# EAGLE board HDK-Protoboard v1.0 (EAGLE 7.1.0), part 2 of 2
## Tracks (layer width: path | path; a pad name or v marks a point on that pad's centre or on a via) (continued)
N$793  (via drill 0.89 pad 1.65)
  other vias: 63.88,62.87
N$794  (via drill 0.89 pad 1.65)
  other vias: 61.34,62.87
N$795  (via drill 0.89 pad 1.65)
  other vias: 63.88,60.33
N$796  (via drill 0.89 pad 1.65)
  other vias: 66.42,60.33
N$797  (via drill 0.89 pad 1.65)
  other vias: 63.88,57.79
N$798  (via drill 0.89 pad 1.65)
  other vias: 64.01,55.25
N$799  (via drill 0.89 pad 1.65)
  other vias: 66.42,55.25
N$800  (via drill 0.89 pad 1.65)
  other vias: 63.88,52.71
N$801  (via drill 0.89 pad 1.65)
  other vias: 61.34,52.71
N$802  (via drill 0.89 pad 1.65)
  other vias: 63.88,50.17
N$803  (via drill 0.89 pad 1.65)
  other vias: 66.42,50.17
N$804  (via drill 0.89 pad 1.65)
  other vias: 63.88,47.63
N$805  (via drill 0.89 pad 1.65)
  other vias: 61.34,47.63
N$806  (via drill 0.89 pad 1.65)
  other vias: 63.88,45.09
N$807  (via drill 0.89 pad 1.65)
  other vias: 66.42,45.09
N$808  (via drill 0.89 pad 1.65)
  other vias: 61.34,42.55
N$809  (via drill 0.89 pad 1.65)
  other vias: 63.88,42.55
N$810  (via drill 0.89 pad 1.65)
  other vias: 63.88,40.01
N$811  (via drill 0.89 pad 1.65)
  other vias: 66.42,40.01
N$812  (via drill 0.89 pad 1.65)
  other vias: 63.88,37.47
N$813  (via drill 0.89 pad 1.65)
  other vias: 63.88,34.93
N$814  (via drill 0.89 pad 1.65)
  other vias: 66.42,34.93
N$815  (via drill 0.89 pad 1.65)
  other vias: 61.34,32.39
N$816  (via drill 0.89 pad 1.65)
  other vias: 63.88,32.39
N$817  (via drill 0.89 pad 1.65)
  other vias: 63.88,29.85
N$818  (via drill 0.89 pad 1.65)
  other vias: 66.42,29.85
N$819  (via drill 0.89 pad 1.65)
  other vias: 61.34,27.31
N$820  (via drill 0.89 pad 1.65)
  other vias: 63.88,27.31
N$821  (via drill 0.89 pad 1.65)
  other vias: 63.88,24.77
N$822  (via drill 0.89 pad 1.65)
  other vias: 66.42,24.77
N$823  (via drill 0.89 pad 1.65)
  other vias: 61.34,22.23
N$824  (via drill 0.89 pad 1.65)
  other vias: 63.88,22.23
N$825  (via drill 0.89 pad 1.65)
  other vias: 63.88,19.69
N$826  (via drill 0.89 pad 1.65)
  other vias: 66.42,19.69
N$827  (via drill 0.89 pad 1.65)
  other vias: 61.34,17.15
N$828  (via drill 0.89 pad 1.65)
  other vias: 63.88,17.15
N$829  (via drill 0.89 pad 1.65)
  other vias: 61.34,12.07
N$830  (via drill 0.89 pad 1.65)
  other vias: 63.88,12.07
N$831  (via drill 0.89 pad 1.65)
  other vias: 63.88,14.61
N$832  (via drill 0.89 pad 1.65)
  other vias: 66.42,14.61
N$833  (via drill 0.89 pad 1.65)
  other vias: 63.88,9.53
N$834  (via drill 0.89 pad 1.65)
  other vias: 66.42,9.53
N$835  (via drill 0.89 pad 1.65)
  other vias: 61.34,6.99
N$836  (via drill 0.89 pad 1.65)
  other vias: 63.88,6.99
N$837  (via drill 0.89 pad 1.65)
  other vias: 63.88,4.45
N$838  (via drill 0.89 pad 1.65)
  other vias: 66.42,4.45
N$839  (via drill 0.89 pad 1.65)
  other vias: 61.34,1.91
N$840  (via drill 0.89 pad 1.65)
  other vias: 63.88,1.91
N$841
  Top 0.406: 43.56,9.53 43.56,1.91
N$842  (via drill 0.89 pad 1.65)
  other vias: 25.02,19.31
N$843  (via drill 0.89 pad 1.65)
  other vias: 27.56,19.31
N$844
  Top 0.406: 43.56,19.69 43.56,12.07
N$845  (via drill 0.89 pad 1.65)
  other vias: 25.02,16.77
N$846  (via drill 0.89 pad 1.65)
  other vias: 27.56,16.77
N$847
  Top 0.406: 43.56,29.85 43.56,22.23
N$848  (via drill 0.89 pad 1.65)
  other vias: 25.02,14.23
N$849  (via drill 0.89 pad 1.65)
  other vias: 27.56,14.23
N$850
  Top 0.406: 43.56,40.01 43.56,32.39
N$851  (via drill 0.89 pad 1.65)
  other vias: 25.02,11.69
N$852  (via drill 0.89 pad 1.65)
  other vias: 27.56,11.69
N$853
  Top 0.406: 43.56,50.17 43.56,42.55
N$854  (via drill 0.89 pad 1.65)
  other vias: 25.02,9.15
N$855  (via drill 0.89 pad 1.65)
  other vias: 27.56,9.15
N$856
  Top 0.406: 43.56,60.33 43.56,52.71
N$857  (via drill 0.89 pad 1.65)
  other vias: 25.02,6.61
N$858  (via drill 0.89 pad 1.65)
  other vias: 27.56,6.61
N$859
  Top 0.406: 43.56,70.49 43.56,62.87
N$860  (via drill 0.89 pad 1.65)
  other vias: 25.02,4.07
N$861  (via drill 0.89 pad 1.65)
  other vias: 27.56,4.07
N$862
  Top 0.406: 43.56,80.65 43.56,73.03
N$863  (via drill 0.89 pad 1.65)
  other vias: 25.02,1.53
N$864  (via drill 0.89 pad 1.65)
  other vias: 27.56,1.53
N$865
  Top 0.406: 46.1,9.53 46.1,1.91
N$866
  Top 0.406: 46.1,19.69 46.1,12.07
N$867
  Top 0.406: 46.1,29.85 46.1,22.23
N$868
  Top 0.406: 46.1,40.01 46.1,32.39
N$869
  Top 0.406: 46.1,50.17 46.1,42.55
N$870
  Top 0.406: 46.1,60.33 46.1,52.71
N$871
  Top 0.406: 46.1,70.49 46.1,62.87
N$872
  Top 0.406: 46.1,80.65 46.1,73.03
N$873
  Top 0.406: 48.64,9.53 48.64,1.91
N$874
  Top 0.406: 48.64,19.69 48.64,12.07
N$875
  Top 0.406: 48.64,29.85 48.64,22.23
N$876
  Top 0.406: 48.64,40.01 48.64,32.39
N$877
  Top 0.406: 48.64,50.17 48.64,42.55
N$878
  Top 0.406: 48.64,60.33 48.64,52.71
N$879
  Top 0.406: 48.64,70.49 48.64,62.87
N$880
  Top 0.406: 48.64,80.65 48.64,73.03
N$881
  Top 0.406: 51.18,9.53 51.18,1.91
N$882
  Top 0.406: 51.18,19.69 51.18,12.07
N$883
  Top 0.406: 51.18,29.85 51.18,22.23
N$884
  Top 0.406: 51.18,40.01 51.18,32.39
N$885
  Top 0.406: 51.18,50.17 51.18,42.55
N$886
  Top 0.406: 51.18,60.33 51.18,52.71
N$887
  Top 0.406: 51.18,70.49 51.18,62.87
N$888
  Top 0.406: 51.18,80.65 51.18,73.03
N$889
  Top 0.406: 53.72,9.53 53.72,1.91
N$890
  Top 0.406: 53.72,19.69 53.72,12.07
N$891
  Top 0.406: 53.72,29.85 53.72,22.23
N$892
  Top 0.406: 53.72,40.01 53.72,32.39
N$893
  Top 0.406: 53.72,50.17 53.72,42.55
N$894
  Top 0.406: 53.72,60.33 53.72,52.71
N$895
  Top 0.406: 53.72,70.49 53.72,62.87
N$896
  Top 0.406: 53.72,80.65 53.72,73.03
N$897
  Top 0.406: 56.26,9.53 56.26,1.91
N$898
  Top 0.406: 56.26,19.69 56.26,12.07
N$899
  Top 0.406: 56.26,29.85 56.26,22.23
N$900
  Top 0.406: 56.26,40.01 56.26,32.39
N$901
  Top 0.406: 56.26,50.17 56.26,42.55
N$902
  Top 0.406: 56.26,60.33 56.26,52.71
N$903
  Top 0.406: 56.26,70.49 56.26,62.87
N$904
  Top 0.406: 56.26,80.65 56.26,73.03
N$905
  Top 0.406: 58.8,9.53 58.8,1.91
N$906
  Top 0.406: 58.8,19.69 58.8,12.07
N$907
  Top 0.406: 58.8,29.85 58.8,22.23
N$908
  Top 0.406: 58.8,40.01 58.8,32.39
N$909
  Top 0.406: 58.8,50.17 58.8,42.55
N$910
  Top 0.406: 58.8,60.33 58.8,52.71
N$911
  Top 0.406: 58.8,70.49 58.8,62.87
N$912
  Top 0.406: 58.8,80.65 58.8,73.03
N$913
  Top 0.406: 61.34,9.53 61.34,1.91
N$914
  Top 0.406: 61.34,19.69 61.34,12.07
N$915
  Top 0.406: 61.34,29.85 61.34,22.23
N$916
  Top 0.406: 61.34,40.01 61.34,32.39
N$917
  Top 0.406: 61.34,50.17 61.34,42.55
N$918
  Top 0.406: 61.34,60.33 61.34,52.71
N$919
  Top 0.406: 61.34,70.49 61.34,62.87
N$920
  Top 0.406: 61.34,80.65 61.34,73.03
N$921
  Top 0.406: 63.88,9.53 63.88,1.91
N$922
  Top 0.406: 63.88,19.69 63.88,12.07
N$923
  Top 0.406: 63.88,29.85 63.88,22.23
N$924
  Top 0.406: 63.88,40.01 63.88,32.39
N$925
  Top 0.406: 63.88,50.17 63.88,42.55
N$926
  Top 0.406: 63.88,60.33 63.88,52.71
N$927
  Top 0.406: 63.88,70.49 63.88,62.87
N$928
  Top 0.406: 63.88,80.65 63.88,73.03
N$929
  Top 0.406: 66.42,9.53 66.42,1.91
N$930
  Top 0.406: 66.42,19.69 66.42,12.07
N$931
  Top 0.406: 66.42,29.85 66.42,22.23
N$932
  Top 0.406: 66.42,40.01 66.42,32.39
N$933
  Top 0.406: 66.42,50.17 66.42,42.55
N$934
  Top 0.406: 66.42,60.33 66.42,52.71
N$935
  Top 0.406: 66.42,70.49 66.42,62.87
N$936
  Top 0.406: 66.42,80.65 66.42,73.03
N$937
  Top 0.406: 68.96,9.53 68.96,1.91
N$938
  Top 0.406: 68.96,19.69 68.96,12.07
N$939
  Top 0.406: 68.96,29.85 68.96,22.23
N$940
  Top 0.406: 68.96,40.01 68.96,32.39
N$941
  Top 0.406: 68.96,50.17 68.96,42.55
N$942
  Top 0.406: 68.96,60.33 68.96,52.71
N$943
  Top 0.406: 68.96,70.49 68.96,62.87
N$944
  Top 0.406: 68.96,80.65 68.96,73.03
N$945
  Top 0.406: 71.5,9.53 71.5,1.91
N$946
  Top 0.406: 71.5,19.69 71.5,12.07
N$947
  Top 0.406: 71.5,29.85 71.5,22.23
N$948
  Top 0.406: 71.5,40.01 71.5,32.39
N$949
  Top 0.406: 71.5,50.17 71.5,42.55
N$950
  Top 0.406: 71.5,60.33 71.5,52.71
N$951
  Top 0.406: 71.5,70.49 71.5,62.87
N$952
  Top 0.406: 71.5,80.65 71.5,73.03
N$953
  Top 0.406: 74.04,9.53 74.04,1.91
N$954
  Top 0.406: 74.04,19.69 74.04,12.07
N$955
  Top 0.406: 74.04,29.85 74.04,22.23
N$956
  Top 0.406: 74.04,40.01 74.04,32.39
N$957
  Top 0.406: 74.04,50.17 74.04,42.55
N$958
  Top 0.406: 74.04,60.33 74.04,52.71
N$959
  Top 0.406: 74.04,70.49 74.04,62.87
N$960
  Top 0.406: 74.04,80.65 74.04,73.03
N$961
  Top 0.406: 76.58,9.53 76.58,1.91
N$962
  Top 0.406: 76.58,19.69 76.58,12.07
N$963
  Top 0.406: 76.58,29.85 76.58,22.23
N$964
  Top 0.406: 76.58,40.01 76.58,32.39
N$965
  Top 0.406: 76.58,50.17 76.58,42.55
N$966
  Top 0.406: 76.58,60.33 76.58,52.71
N$967
  Top 0.406: 76.58,70.49 76.58,62.87
N$968
  Top 0.406: 76.58,80.65 76.58,73.03
N$969
  Top 0.406: 79.12,9.53 79.12,1.91
N$970
  Top 0.406: 79.12,19.69 79.12,12.07
N$971
  Top 0.406: 79.12,29.85 79.12,22.23
N$972
  Top 0.406: 79.12,40.01 79.12,32.39
N$973
  Top 0.406: 79.12,50.17 79.12,42.55
N$974
  Top 0.406: 79.12,60.33 79.12,52.71
N$975
  Top 0.406: 79.12,70.49 79.12,62.87
N$976
  Top 0.406: 79.12,80.65 79.12,73.03
N$977
  Top 0.406: 81.66,9.53 81.66,1.91
N$978
  Top 0.406: 81.66,19.69 81.66,12.07
N$979
  Top 0.406: 81.66,29.85 81.66,22.23
N$980
  Top 0.406: 81.66,40.01 81.66,32.39
N$981
  Top 0.406: 81.66,50.17 81.66,42.55
N$982
  Top 0.406: 81.66,60.33 81.66,52.71
N$983
  Top 0.406: 81.66,70.49 81.66,62.87
N$984
  Top 0.406: 81.66,80.65 81.66,73.03
N$985
  Top 0.406: 84.2,9.53 84.2,1.91
N$986
  Top 0.406: 84.2,19.69 84.2,12.07
N$987
  Top 0.406: 84.2,29.85 84.2,22.23
N$988
  Top 0.406: 84.2,40.01 84.2,32.39
N$989
  Top 0.406: 84.2,50.17 84.2,42.55
N$990
  Top 0.406: 84.2,60.33 84.2,52.71
N$991
  Top 0.406: 84.2,70.49 84.2,62.87
N$992
  Top 0.406: 84.2,80.65 84.2,73.03
N$993
  Top 0.406: 86.74,9.53 86.74,1.91
N$994
  Top 0.406: 86.74,19.69 86.74,12.07
N$995
  Top 0.406: 86.74,29.85 86.74,22.23
N$996
  Top 0.406: 86.74,40.01 86.74,32.39
N$997
  Top 0.406: 86.74,50.17 86.74,42.55
N$998
  Top 0.406: 86.74,60.33 86.74,52.71
N$999
  Top 0.406: 86.74,70.49 86.74,62.87
N$1000
  Top 0.406: 86.74,80.65 86.74,73.03
N$1001
  Top 0.406: 89.28,9.53 89.28,1.91
N$1002
  Top 0.406: 89.28,19.69 89.28,12.07
N$1003
  Top 0.406: 89.28,29.85 89.28,22.23
N$1004
  Top 0.406: 89.28,40.01 89.28,32.39
N$1005
  Top 0.406: 89.28,50.17 89.28,42.55
N$1006
  Top 0.406: 89.28,60.33 89.28,52.71
N$1007
  Top 0.406: 89.28,70.49 89.28,62.87
N$1008
  Top 0.406: 89.28,80.65 89.28,73.03
N$1009
  Top 0.406: 91.82,9.53 91.82,1.91
N$1010
  Top 0.406: 91.82,19.69 91.82,12.07
N$1011
  Top 0.406: 91.82,29.85 91.82,22.23
N$1012
  Top 0.406: 91.82,40.01 91.82,32.39
N$1013
  Top 0.406: 91.82,50.17 91.82,42.55
N$1014
  Top 0.406: 91.82,60.33 91.82,52.71
N$1015
  Top 0.406: 91.82,70.49 91.82,62.87
N$1016
  Top 0.406: 91.82,80.65 91.82,73.03
N$1017
  Top 0.406: 94.36,9.53 94.36,1.91
N$1018
  Top 0.406: 94.36,19.69 94.36,12.07
N$1019
  Top 0.406: 94.36,29.85 94.36,22.23
N$1020
  Top 0.406: 94.36,40.01 94.36,32.39
N$1021
  Top 0.406: 94.36,50.17 94.36,42.55
N$1022
  Top 0.406: 94.36,60.33 94.36,52.71
N$1023
  Top 0.406: 94.36,70.49 94.36,62.87
N$1024
  Top 0.406: 94.36,80.65 94.36,73.03
N$1025
  Top 0.406: 96.9,9.53 96.9,1.91
N$1026
  Top 0.406: 96.9,19.69 96.9,12.07
N$1027
  Top 0.406: 96.9,29.85 96.9,22.23
N$1028
  Top 0.406: 96.9,40.01 96.9,32.39
N$1029
  Top 0.406: 96.9,50.17 96.9,42.55
N$1030
  Top 0.406: 96.9,60.33 96.9,52.71
N$1031
  Top 0.406: 96.9,70.49 96.9,62.87
N$1032
  Top 0.406: 96.9,80.65 96.9,73.03
N$1033
  Top 0.406: 99.44,9.53 99.44,1.91
N$1034
  Top 0.406: 99.44,19.69 99.44,12.07
N$1035
  Top 0.406: 99.44,29.85 99.44,22.23
N$1036
  Top 0.406: 99.44,40.01 99.44,32.39
N$1037
  Top 0.406: 99.44,50.17 99.44,42.55
N$1038
  Top 0.406: 99.44,60.33 99.44,52.71
N$1039
  Top 0.406: 99.44,70.49 99.44,62.87
N$1040
  Top 0.406: 99.44,80.65 99.44,73.03
N$1041
  Top 0.406: 101.98,9.53 101.98,1.91
N$1042
  Top 0.406: 101.98,19.69 101.98,12.07
N$1043
  Top 0.406: 101.98,29.85 101.98,22.23
N$1044
  Top 0.406: 101.98,40.01 101.98,32.39
N$1045
  Top 0.406: 101.98,50.17 101.98,42.55
N$1046
  Top 0.406: 101.98,60.33 101.98,52.71
N$1047
  Top 0.406: 101.98,70.49 101.98,62.87
N$1048
  Top 0.406: 101.98,80.65 101.98,73.03
N$1049
  Top 0.406: 104.52,9.53 104.52,1.91
N$1050
  Top 0.406: 104.52,19.69 104.52,12.07
N$1051
  Top 0.406: 104.52,29.85 104.52,22.23
N$1052
  Top 0.406: 104.52,40.01 104.52,32.39
N$1053
  Top 0.406: 104.52,50.17 104.52,42.55
N$1054
  Top 0.406: 104.52,60.33 104.52,52.71
N$1055
  Top 0.406: 104.52,70.49 104.52,62.87
N$1056
  Top 0.406: 104.52,80.65 104.52,73.03
VIN1  (via drill 0.89 pad 1.65)
  Top 0.61: J2.+ 11.11,47.06 16.76,52.71 v22.48,52.71 v25.02,52.71 v27.56,52.71
VIN2  (via drill 0.89 pad 1.65)
  Top 0.61: v25.02,31.63 v22.48,31.63 8.78,31.63 J3.+ | 25.15,31.63 v25.02,31.63 | v25.02,31.63 v27.56,31.63
VUSB  (via drill 0.89 pad 1.65)
  Top 0.406: J1.1 5.36,74.2 5.59,74.42
  Top 0.61: 5.59,74.42 7.87,76.71 v22.48,76.71 v25.02,76.71 v27.56,76.71

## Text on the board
tPlace: A | B | C | D | E | F | G | H | I | J | K | L | M | N | O | P | Q | R | S | T | U | V | W | X | Y | Z | 1 | 5V | 2 | VUSB | 3 | D- | 4 | D+ | 5 | GND | 6 | 7 | 8 | 9 | 10 | 9-12V | 11 | VIN | 12 | GND | 13 | 14 | 15 | opl.seeed.cc | 16 | 17 | 18 | 19 | 20 | VIN | GND | 21 | 22 | 23 | 24 | A1 | 25 | 26 | A2 | A3 | 27 | 28 | A4 | A5 | 29 | A6 | 30 | A7 | 31 | A8 | 32
bPlace: A | B | C | D | E | F | G | H | I | J | K | L | M | N | O | P | Q | R | S | T | U | V | W | X | Y | Z | 1 | 2 | 3 | 4 | 5 | 6 | 7 | 8 | 9 | HDK-Protoboard v1.0 | 10 | 11 | 12 | 13 | 14 | 15 | 16 | 17 | 18 | 19 | 20 | 21 | 22 | 23 | 24 | 25 | 26 | 27 | 28 | 29 | 30 | 31 | 32
dxf: V-CUT | V-CUT | V-CUT | V-CUT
